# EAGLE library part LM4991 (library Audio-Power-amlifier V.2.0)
The LM4991 is a mono bridged audio power amplifier capable of delivering 3W of continuous average power into a 3Ω load with less than 10% THD when powered by a 5V power supply (see Note below). To conserve power in portable applications, the LM4991's micropower shutdown mode (ISD = 0.1μA, typ) is activated when VDD is applied to the SHUTDOWN pin.
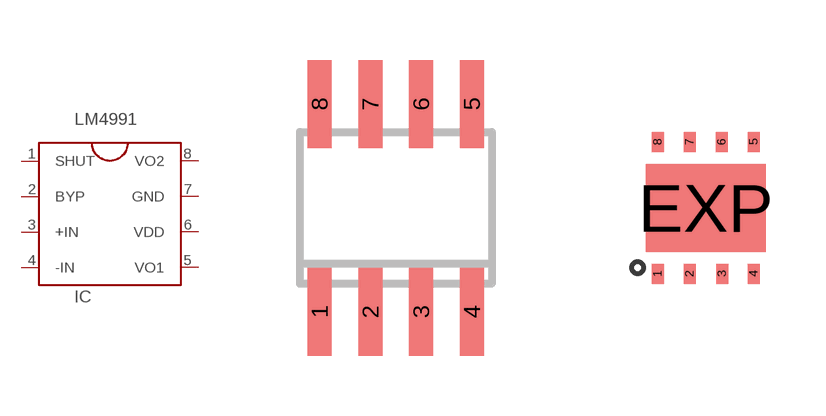
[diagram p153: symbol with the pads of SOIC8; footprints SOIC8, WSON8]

Designator prefix IC

## LM4991LM4991MAX/NOPB  [SOIC8]
1  SHUT  in
2  BYP  in
3  +IN  in
4  -IN  in
5  VO1  out
6  VDD  pwr
7  GND  pwr
8  VO2  out

## LM4991LM4991LDX/NOPB  [WSON8]
Pads as for SOIC8

## Footprint SOIC8 (pad centres in mm)
Small Outline IC
smd 0.6 x 2.2: 1 -1.905,-2.6; 2 -0.635,-2.6; 3 0.635,-2.6; 4 1.905,-2.6; 5 1.905,2.6; 6 0.635,2.6; 7 -0.635,2.6; 8 -1.905,2.6

## Footprint WSON8 (pad centres in mm)
LLP4x4 body. http://www.ti.com/sc/docs/package/guide.htm
smd 0.3 x 0.5: 1 -1.2,-1.65; 2 -0.4,-1.65; 3 0.41,-1.65; 4 1.2,-1.65; 5 1.2,1.65; 6 0.4,1.65; 7 -0.4,1.65; 8 -1.2,1.65
smd 3 x 2.2: EXP 0,0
